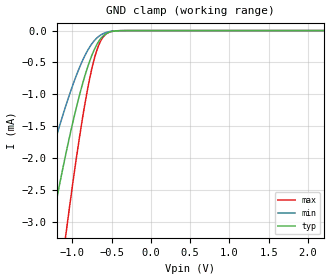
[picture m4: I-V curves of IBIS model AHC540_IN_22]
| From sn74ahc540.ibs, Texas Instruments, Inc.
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[Model]   AHC540_IN_22
Model_type  Input
Vinl = 0.5
Vinh = 1.5
| variable   typ   min   max
C_comp   0.59pF   0.54pF   0.66pF
[Temperature Range]   40   100   -40
| Ambient temperature   25   85   -40
[Voltage range]   2.2   2   2.4
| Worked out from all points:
|   GND clamp passes 1 mA (typ) near -0.91 V on its own axis
[GND Clamp]
| AHC540_IN_22
|   Voltage   I(typ)   I(min)   I(max)
-5V       -39.52mA   -26.01mA   -50.56mA
-1.555V   -5.15mA    -3.294mA   -8.098mA
-1.505V   -4.772mA   -3.046mA   -7.55mA
-1.28V    -3.176mA   -1.997mA   -5.16mA
-1.075V   -1.894mA   -1.151mA   -3.138mA
-910mV    -1.022mA   -586uA     -1.69mA
-775mV    -468.1uA   -251.6uA   -732.6uA
-680mV    -203.9uA   -109.1uA   -283.9uA
-625mV    -107uA     -59.91uA   -134uA
-565mV    -45.17uA   -27.54uA   -48.8uA
-385mV    -1.717uA   -1.229uA   -925.9nA
2.2V      1.234nA    466.5pA    2.192nA
